[IBIS ver]   3.2
[File name]   7448_25v_r3.ibs
[File Rev]   3.0
[Date]   12/19/05
[Source]   Simulation-based IO data.
[Notes]   Per-pin package parasitics based on board file
|   including Er values, stackup, and trace dimensions.
|   Pin resistance values based on resistance at DC
 Revision history:
   Rev 1: initial release
   IBIS Simulation Notes:
   -  Passes IBIS Checker 3.2.9 and ICX Checker
   -  Runs in Hyperlynx and HSPICE.
   -  If IBIS produces spurious spike in HSPICE,
   try setting  ramp_rwf=0.
 11/11/05 - ME - Rev 2
   Revised model files to prevent spurious spikes in SPICE
   Revised C_comp values
   Changed pin A12 name to "DFS2_B" (to match documentation)
   Passes ICX checker
 12/19/05 - Signal Integrity Software Inc. (SiSoft) - Rev. 3.0
   Added per-pin package parasitics
[Disclaimer]   This information is for modeling purposes only
|   and is not guaranteed.
[Component]   7448
[Manufacturer]   Freescale, Inc.
[Package]
|variable   typ   min   max
R_pkg   0.485   NA   NA
L_pkg   5.506nH   NA   NA
C_pkg   0.917pF   NA   NA
[Pin]  signal_name   model_name   R_pin  L_pin   C_pin
E11   A(0)   busio_25_rev1_1   0.513  6.178nH  0.899pF
H1   A(1)   busio_25_rev1_1   0.481  4.541nH  1.132pF
D12   A(10)   busio_25_rev1_1   0.617  7.396nH  1.080pF
L3   A(11)   busio_25_rev1_1   0.365  3.583nH  0.832pF
G4   A(12)   busio_25_rev1_1   0.611  7.552nH  1.019pF
T2   A(13)   busio_25_rev1_1   0.729  8.461nH  1.267pF
F4   A(14)   busio_25_rev1_1   0.723  8.933nH  1.205pF
V1   A(15)   busio_25_rev1_1   0.899  10.923nH 1.578pF
J4   A(16)   busio_25_rev1_1   0.297  2.921nH  0.678pF
R2   A(17)   busio_25_rev1_1   0.592  6.579nH  1.162pF
K5   A(18)   busio_25_rev1_1   0.186  1.754nH  0.437pF
W2   A(19)   busio_25_rev1_1   0.877  9.292nH  1.828pF
C11   A(2)   busio_25_rev1_1   0.533  6.365nH  0.932pF
J2   A(20)   busio_25_rev1_1   0.378  4.663nH  0.629pF
K4   A(21)   busio_25_rev1_1   0.248  3.061nH  0.413pF
N4   A(22)   busio_25_rev1_1   0.256  2.415nH  0.602pF
J3   A(23)   busio_25_rev1_1   0.314  3.878nH  0.523pF
M5   A(24)   busio_25_rev1_1   0.212  2.371nH  0.366pF
P5   A(25)   busio_25_rev1_1   0.330  3.408nH  0.623pF
N3   A(26)   busio_25_rev1_1   0.310  3.831nH  0.517pF
T1   A(27)   busio_25_rev1_1   0.712  8.619nH  1.249pF
V2   A(28)   busio_25_rev1_1   0.801  9.879nH  1.386pF
U1   A(29)   busio_25_rev1_1   0.925  10.235nH 1.873pF
G3   A(3)   busio_25_rev1_1   0.613  7.567nH  1.021pF
N5   A(30)   busio_25_rev1_1   0.215  2.600nH  0.378pF
W1   A(31)   busio_25_rev1_1   0.872  9.285nH  1.806pF
B12   A(32)   busio_25_rev1_1   0.673  7.906nH  1.173pF
C4   A(33)   busio_25_rev1_1   0.639  7.239nH  1.259pF
G10   A(34)   busio_25_rev1_1   0.261  3.011nH  0.453pF
B11   A(35)   busio_25_rev1_1   0.808  9.743nH  1.417pF
F10   A(4)   busio_25_rev1_1   0.616  7.134nH  1.070pF
L2   A(5)   busio_25_rev1_1   0.418  4.913nH  0.728pF
D11   A(6)   busio_25_rev1_1   0.587  6.997nH  1.026pF
D1   A(7)   busio_25_rev1_1   0.636  7.850nH  1.059pF
C10   A(8)   busio_25_rev1_1   0.792  9.629nH  1.391pF
G2   A(9)   busio_25_rev1_1   0.507  4.794nH  1.195pF
R1   AACK_B   busio_25_rcvr_rev1   0.554  5.651nH  1.208pF
C1   AP(0)   busio_25_rev1_1   0.942  11.235nH 1.665pF
E3   AP(1)   busio_25_rev1_1   0.770  8.400nH  1.584pF
H6   AP(2)   busio_25_rev1_1   0.128  1.586nH  0.214pF
F5   AP(3)   busio_25_rev1_1   0.545  6.101nH  1.089pF
G7   AP(4)   busio_25_rev1_1   0.124  1.405nH  0.214pF
N2   ARTRY_B   busio_25_rev1_1   0.597  6.499nH  1.231pF
M1   BG_B   busio_25_rcvr_rev1   0.639  7.897nH  1.066pF
G9   BMODE_B(0)   busio_25_rcvr_rev1   0.456  5.634nH  0.770pF
F8   BMODE_B(1)   busio_25_rcvr_rev1   0.158  1.809nH  0.273pF
D2   BR_B   busio_25_rev1_1   0.689  8.509nH  1.148pF
B7   BVSEL0   busio_25_rcvr_rev1   0.478  4.517nH  1.126pF
E10   BVSEL1   busio_25_rcvr_rev1   0.318  3.004nH  0.749pF
J1   CI_B   busio_25_rev1_1   0.810  10.001nH 1.350pF
A3   CKSTP_IN_B   busio_25_rcvr_rev1   0.610  7.536nH  1.017pF
B1   CKSTP_OUT_B   busio_25_rev1_1   0.819  7.737nH  1.929pF
H2   CLK_OUT   busio_25_rev1_1   0.367  3.472nH  0.865pF
R15   D(0)   busio_25_rev1_1   0.257  3.171nH  0.428pF
W15   D(1)   busio_25_rev1_1   0.577  5.454nH  1.360pF
T13   D(10)   busio_25_rev1_1   0.290  3.439nH  0.506pF
P13   D(11)   busio_25_rev1_1   0.165  1.825nH  0.335pF
U14   D(12)   busio_25_rev1_1   0.311  3.695nH  0.555pF
W14   D(13)   busio_25_rev1_1   0.519  6.189nH  0.908pF
R12   D(14)   busio_25_rev1_1   0.174  1.646nH  0.410pF
T12   D(15)   busio_25_rev1_1   0.242  2.283nH  0.569pF
W12   D(16)   busio_25_rev1_1   0.481  5.809nH  0.844pF
V12   D(17)   busio_25_rev1_1   0.357  3.376nH  0.842pF
N11   D(18)   busio_25_rev1_1   0.083  0.903nH  0.143pF
N10   D(19)   busio_25_rev1_1   0.052  0.566nH  0.108pF
T14   D(2)   busio_25_rev1_1   0.350  3.304nH  0.824pF
R11   D(20)   busio_25_rev1_1   0.181  2.020nH  0.312pF
U11   D(21)   busio_25_rev1_1   0.303  3.525nH  0.527pF
W11   D(22)   busio_25_rev1_1   0.489  4.625nH  1.153pF
T11   D(23)   busio_25_rev1_1   0.194  2.402nH  0.324pF
R10   D(24)   busio_25_rev1_1   0.145  1.370nH  0.341pF
N9   D(25)   busio_25_rev1_1   0.187  1.430nH  0.301pF
P10   D(26)   busio_25_rev1_1   0.078  0.733nH  0.183pF
U10   D(27)   busio_25_rev1_1   0.254  3.140nH  0.424pF
R9   D(28)   busio_25_rev1_1   0.150  1.853nH  0.250pF
W10   D(29)   busio_25_rev1_1   0.444  5.265nH  0.776pF
V16   D(3)   busio_25_rev1_1   0.439  4.145nH  1.033pF
U9   D(30)   busio_25_rev1_1   0.282  2.667nH  0.665pF
V9   D(31)   busio_25_rev1_1   0.406  5.008nH  0.676pF
W5   D(32)   busio_25_rev1_1   0.496  6.123nH  0.826pF
U6   D(33)   busio_25_rev1_1   0.423  5.017nH  0.739pF
T5   D(34)   busio_25_rev1_1   0.351  3.316nH  0.827pF
U5   D(35)   busio_25_rev1_1   0.507  6.055nH  0.886pF
W7   D(36)   busio_25_rev1_1   0.494  5.984nH  0.867pF
R6   D(37)   busio_25_rev1_1   0.266  2.511nH  0.626pF
P7   D(38)   busio_25_rev1_1   0.357  3.866nH  0.612pF
V6   D(39)   busio_25_rev1_1   0.399  4.930nH  0.665pF
W16   D(4)   busio_25_rev1_1   0.604  7.239nH  1.058pF
P17   D(40)   busio_25_rev1_1   0.529  5.905nH  1.030pF
R19   D(41)   busio_25_rev1_1   0.651  7.709nH  1.211pF
V18   D(42)   busio_25_rev1_1   0.543  6.184nH  1.028pF
R18   D(43)   busio_25_rev1_1   0.534  6.448nH  0.936pF
V19   D(44)   busio_25_rev1_1   0.591  5.587nH  1.393pF
T19   D(45)   busio_25_rev1_1   0.652  7.816nH  1.142pF
U19   D(46)   busio_25_rev1_1   0.542  5.118nH  1.276pF
W19   D(47)   busio_25_rev1_1   0.685  8.462nH  1.142pF
U18   D(48)   busio_25_rev1_1   0.514  6.343nH  0.856pF
W17   D(49)   busio_25_rev1_1   0.577  6.778nH  1.045pF
T15   D(5)   busio_25_rev1_1   0.352  4.207nH  0.616pF
W18   D(50)   busio_25_rev1_1   0.625  7.724nH  1.042pF
T16   D(51)   busio_25_rev1_1   0.338  3.196nH  0.797pF
T18   D(52)   busio_25_rev1_1   0.493  6.092nH  0.822pF
T17   D(53)   busio_25_rev1_1   0.389  4.804nH  0.648pF
W3   D(54)   busio_25_rev1_1   0.751  9.131nH  1.318pF
V17   D(55)   busio_25_rev1_1   0.524  6.468nH  0.873pF
U4   D(56)   busio_25_rev1_1   0.491  5.848nH  0.858pF
U8   D(57)   busio_25_rev1_1   0.313  3.862nH  0.521pF
U7   D(58)   busio_25_rev1_1   0.314  2.968nH  0.740pF
R7   D(59)   busio_25_rev1_1   0.188  2.133nH  0.370pF
U15   D(6)   busio_25_rev1_1   0.425  5.119nH  0.745pF
P6   D(60)   busio_25_rev1_1   0.215  2.653nH  0.358pF
R8   D(61)   busio_25_rev1_1   0.181  2.229nH  0.301pF
W8   D(62)   busio_25_rev1_1   0.447  4.229nH  1.054pF
T8   D(63)   busio_25_rev1_1   0.249  3.077nH  0.415pF
P14   D(7)   busio_25_rev1_1   0.219  2.472nH  0.378pF
V13   D(8)   busio_25_rev1_1   0.369  4.553nH  0.614pF
W13   D(9)   busio_25_rev1_1   0.548  6.598nH  0.960pF
M2   DBG_B   busio_25_rcvr_rev1   0.502  6.201nH  0.837pF
A12   DFS2_B   busio_25_rcvr_rev1   0.655  7.937nH  1.149pF
B6   DFS4_B   busio_25_rcvr_rev1   0.597  6.927nH  1.143pF
T3   DP(0)   busio_25_rev1_1   0.418  4.686nH  0.811pF
W4   DP(1)   busio_25_rev1_1   0.684  8.342nH  1.202pF
T4   DP(2)   busio_25_rev1_1   0.426  5.048nH  0.744pF
W9   DP(3)   busio_25_rev1_1   0.458  4.548nH  1.032pF
M6   DP(4)   busio_25_rev1_1   0.280  3.178nH  0.532pF
V3   DP(5)   busio_25_rev1_1   0.590  7.160nH  1.035pF
N8   DP(6)   busio_25_rev1_1   0.127  1.568nH  0.218pF
W6   DP(7)   busio_25_rev1_1   0.615  5.815nH  1.449pF
R3   DRDY_B   busio_25_rev1_1   0.567  6.202nH  0.974pF
G1   DTI(0)   busio_25_rcvr_rev1   0.586  6.104nH  1.255pF
K1   DTI(1)   busio_25_rcvr_rev1   0.806  7.617nH  1.899pF
P1   DTI(2)   busio_25_rcvr_rev1   0.690  8.017nH  1.200pF
N1   DTI(3)   busio_25_rcvr_rev1   0.548  5.350nH  1.255pF
A11   EXT_QUAL   busio_25_rcvr_rev1   0.588  7.035nH  1.029pF
E2   GBL_B   busio_25_rev1_1   0.750  7.903nH  1.573pF
B2   HIT_B   busio_25_rev1_1   0.670  8.274nH  1.117pF
D8   HRESET_B   busio_25_rcvr_rev1   0.301  3.490nH  0.524pF
D4   INT_B   busio_25_rcvr_rev1   0.813  9.470nH  1.415pF
G8   L1_TSTCLK   busio_25_rcvr_rev1   0.208  1.946nH  0.346pF
B3   L2_TSTCLK   busio_25_rcvr_rev1   0.820  8.103nH  1.847pF
E8   LSSD_MODE_B   busio_25_rcvr_rev1   0.251  2.882nH  0.435pF
B10   LVRAM_B   busio_25_rev1_1   0.634  7.834nH  1.057pF
C9   MCP_B   busio_25_rcvr_rev1   0.439  4.145nH  1.033pF
B8   PLL_CFG(0)   busio_25_rcvr_rev1   0.707  8.598nH  1.242pF
C8   PLL_CFG(1)   busio_25_rcvr_rev1   0.698  7.827nH  1.351pF
C7   PLL_CFG(2)   busio_25_rcvr_rev1   0.604  7.239nH  1.058pF
D7   PLL_CFG(3)   busio_25_rcvr_rev1   0.622  7.246nH  1.139pF
A7   PLL_CFG(4)   busio_25_rcvr_rev1   0.740  8.522nH  1.379pF
D10   PLL_CFG(5)   busio_25_rcvr_rev1   0.512  6.327nH  0.854pF
D9   PMON_IN_B   busio_25_rcvr_rev1   0.393  3.712nH  0.925pF
A9   PMON_OUT_B   busio_25_rev1_1   0.576  5.442nH  1.357pF
G5   QACK_B   busio_25_rcvr_rev1   0.309  3.307nH  0.648pF
P4   QREQ_B   busio_25_rev1_1   0.306  2.895nH  0.722pF
E4   SHD0_B   busio_25_rev1_1   0.834  8.235nH  1.880pF
H5   SHD1_B   busio_25_rev1_1   0.198  2.449nH  0.331pF
F9   SMI_B   busio_25_rcvr_rev1   0.332  3.460nH  0.565pF
A2   SRESET_B   busio_25_rcvr_rev1   0.857  8.098nH  2.018pF
A10   SYSCLK   busio_25_rcvr_rev1   0.759  8.367nH  1.504pF
K6   TA_B   busio_25_rcvr_rev1   0.422  4.419nH  0.718pF
E1   TBEN   busio_25_rcvr_rev1   0.765  7.233nH  1.803pF
F11   TBST_B   busio_25_rev1_1   0.369  3.873nH  0.628pF
C6   TCK   busio_25_rcvr_rev1   0.480  5.793nH  0.841pF
B9   TDI   busio_25_rcvr_rev1   0.712  8.792nH  1.186pF
A4   TDO   busio_25_rev1_1   0.976  11.435nH 1.700pF
L1   TEA_B   busio_25_rcvr_rev1   0.577  7.128nH  0.962pF
F1   TMS   busio_25_rcvr_rev1   0.850  10.503nH 1.417pF
A5   TRST_B   busio_25_rcvr_rev1   0.540  6.672nH  0.900pF
G6   TSIZ(0)   busio_25_rev1_1   0.329  3.642nH  0.666pF
F7   TSIZ(1)   busio_25_rev1_1   0.437  5.101nH  0.755pF
E7   TSIZ(2)   busio_25_rev1_1   0.453  5.441nH  0.794pF
L4   TS_B   busio_25_rev1_1   0.283  3.248nH  0.491pF
E5   TT(0)   busio_25_rev1_1   0.341  4.208nH  0.568pF
E6   TT(1)   busio_25_rev1_1   0.413  4.702nH  0.809pF
F6   TT(2)   busio_25_rev1_1   0.310  3.520nH  0.609pF
E9   TT(3)   busio_25_rev1_1   0.512  5.670nH  0.881pF
C5   TT(4)   busio_25_rev1_1   0.458  5.652nH  0.763pF
D3   WT_B   busio_25_rev1_1   1.280  15.810nH 2.133pF
N18   TEMP_ANODE   NC   0.365  4.498nH  0.643pF
N19   TEMP_CATHODE   NC   0.423  5.088nH  0.741pF
| Models and submodels in the file (2): busio_25_rev1_1 (I/O), busio_25_rcvr_rev1 (Input)
